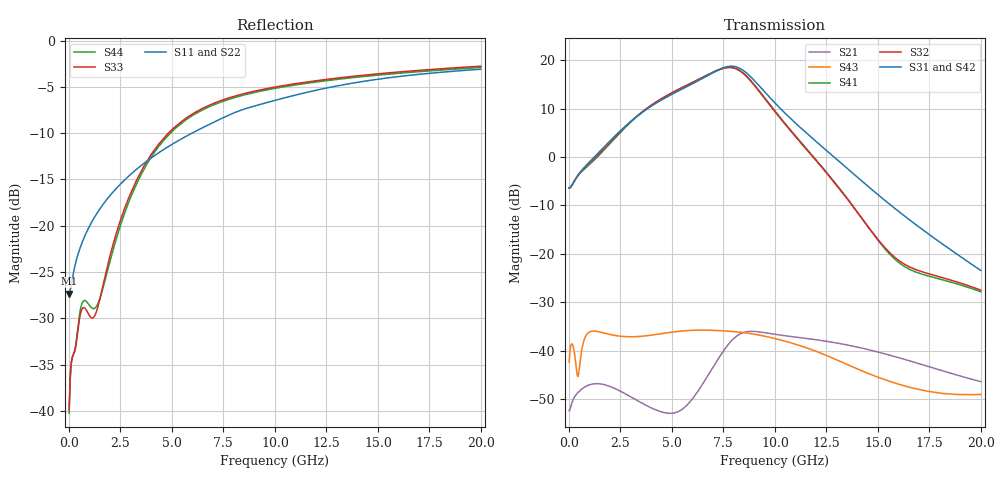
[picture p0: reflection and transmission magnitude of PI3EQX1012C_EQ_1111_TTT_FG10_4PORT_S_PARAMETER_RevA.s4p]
! NPort=4 DATA=2000 NOISE=0 GROUPDELAY=0 COMPLEX_DATAFORMAT=POLAR
! NumOfBlock=1 NumOfParam=0
! .MODEL Smodel S TSTONEFILE=PI3EQX1012C_EQ_1111_TTT_FG10_4PORT_S_PARAMETER_RevA.s4p TYPE=S
!  -- The above .MODEL line can be used for the S element in the netlist.
! The s parameter is extracted from the linear redriver, it is not bi-directional; only s(4,1)s(4,2) and s(3,1)s(3,2)
! should be the insertion loss
!Port definition:
!Port1 = input+
!Port2 = input-
!Port3 = output+
!Port4 = output-
# Hz S MA R  50
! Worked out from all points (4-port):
!   2000 points, 10 MHz to 20 GHz, reference 50 ohm
!   strongest paths, dB at 10 MHz, 5.01 GHz, 10.01 GHz, 15.01 GHz, 20 GHz:
!     S31: -6.4, 13.0, 11.1, -7.8, -23.5
!     S42: -6.4, 13.0, 11.2, -7.6, -23.1
!     S32: -6.4, 13.3, 9.3, -17.1, -27.5
!     S41: -6.4, 13.3, 9.5, -17.2, -27.9
!     S43: -42.4, -36.2, -37.5, -45.5, -49.1
!     S21: -52.4, -53.0, -36.6, -40.3, -46.4
!   lowest |S11| = -27.3 dB at 10 MHz (marker M1), VSWR 1.09, Z = 45.9 - j0.123 ohm
!   |S11| at or under -10 dB: start of sweep to 5.974 GHz
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1e7  0.04301 -178.2  0.002379 1.5  0.0008102 -0.5  0.0008039 -0.5
     0.002388 1.5  0.04109 -178.1  0.000927 -0.5  0.0009197 -0.5
     0.4788 0.5  0.4779 -179.4  0.01016 -4.0  0.007598 -25.7
     0.4774 -179.4  0.4797 0.5  0.007614 -25.8  0.009722 -4.0
5.73e9  0.3059 -123.6  0.002849 56.9  0.0002789 -58.3  0.0002778 -59.3
        0.002724 54.5  0.3108 -122.9  0.0003163 -59.3  0.0003151 -60.2
        5.337 -129.5  5.508 58.6  0.384 -99.3  0.01642 9.8
        5.526 58.8  5.357 -127.6  0.01606 7.2  0.3763 -99.1
7.21e9  0.3703 -124.2  0.008382 69.6  0.0002372 -55.6  0.000235 -56.9
        0.007955 70.7  0.3756 -123.7  0.0002673 -56.8  0.000265 -58.2
        7.865 158.9  7.836 -14.3  0.4665 -110.6  0.0167 -13.2
        7.902 -14.4  7.904 161.0  0.01609 -13.6  0.458 -110.5
8.15e9  0.4126 -125.9  0.01457 43.5  0.0002248 -54.2  0.0002218 -55.7
        0.01413 45.2  0.4184 -125.3  0.0002518 -55.6  0.0002484 -57.1
        8.501 95.4  8.073 -78.6  0.5046 -116.1  0.01586 -26.1
        8.163 -79.0  8.543 97.7  0.01558 -25.7  0.4959 -116.0
9.03e9  0.4439 -127.8  0.016 14.1  0.0002178 -53.8  0.000214 -55.4
        0.01573 15.8  0.4507 -127.3  0.0002426 -55.1  0.0002385 -56.6
        6.078 37.3  5.411 -137.1  0.5337 -120.3  0.01486 -36.5
        5.484 -137.8  6.108 39.8  0.01471 -36.9  0.525 -120.2
1.064e10  0.496 -130.2  0.01417 -14.4  0.0002092 -55.0  0.0002045 -56.5
          0.01408 -13.3  0.5039 -129.8  0.0002317 -55.9  0.0002268 -57.5
          2.642 -32.9  2.001 153.6  0.5767 -126.3  0.01251 -54.3
          2.034 152.2  2.658 -29.8  0.01224 -55.1  0.5676 -126.2
2e10  0.7 -144.7  0.004851 -76.6  0.0001461 -72.3  0.000141 -73.8
      0.004766 -75.6  0.7151 -144.4  0.000162 -72.1  0.0001563 -73.8
      0.06707 99.5  0.04206 27.1  0.7272 -143.5  0.003596 -51.4
      0.04043 25.8  0.07025 104.4  0.003514 -48.7  0.7152 -143.3
